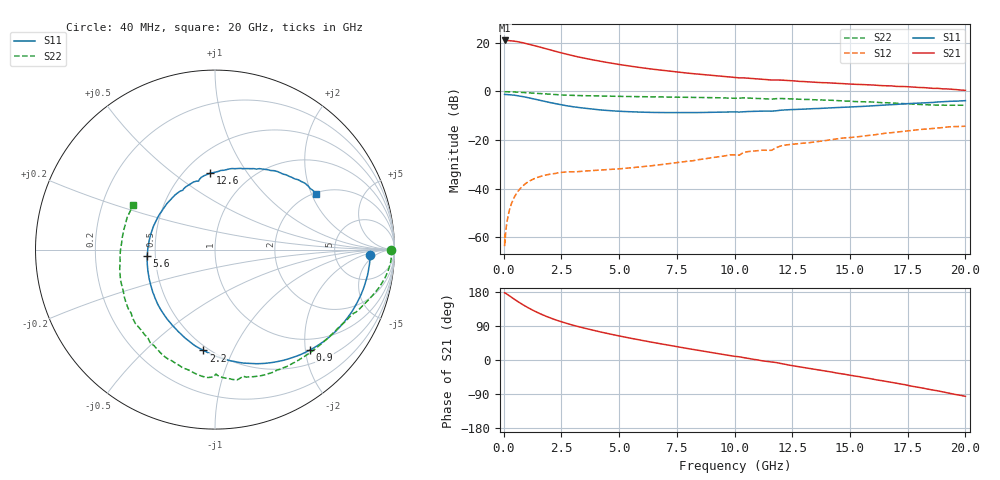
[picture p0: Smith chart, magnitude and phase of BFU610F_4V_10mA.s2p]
! Filename:  P:\Prog\Test\Noise\ATS_data\Testdata_Net\SplitFiles\BFU610_2W_A5_HighFreq_4V_10mA_D.s2p
! Date/Time: Wed 10/Aug/2011 16:57:59
! BFU610_2W_A5_HighFreq_4V_1mA_10mA_Bias4_R.s2p
! MDIF S-parameter v. bias file
! BFU610_2W_A5_HighFreq_4V_1mA_10mA
! Date/time Mon Aug 08 14:12:42 2011
! VAR V_out= 4.0010
! VAR I_out= 10.0000
! VAR V_in= 0.9022
! VAR I_in= 0.0905
! Device data file deembeded for feedlines and parallel
! Original file: \SplitFiles\BFU610_2W_A5_HighFreq_4V_10mA_R.s2p
! Feed-files: PR003V01_101208_Feed1.s2p, PR003V01_101208_Feed2.s2p
! Parallel-file: PR003V01_101208_Par.s2p
# MHz S MA R 50
!  Freq-MHz  S11-mag  S11-arg  S21-mag  S21-arg  S12-mag  S12-arg  S22-mag  S22-arg
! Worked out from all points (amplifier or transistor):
!   167 points, 40 MHz to 20 GHz, reference 50 ohm
!   highest |S21| = 21.0 dB at 40 MHz (marker M1)
!   |S21| within 3 dB of that: start of sweep to 1.673 GHz
!   unconditionally stable (mu >= 1): 3.031 GHz to end of sweep
!   at 550 MHz: K = 0.18, MSG = 31.3 dB, |S12| = -42.1 dB
!   at 4.2 GHz: K = 1.37, MAG = 18.8 dB, |S12| = -32.4 dB
!   at 20 GHz: K = 1.03, MAG = 6.4 dB, |S12| = -14.3 dB
!   S11 on the Smith chart (normalised r, x): 40 MHz: 13, -3; 900 MHz: 0.76, -2.10; 2.2 GHz: 0.47, -0.78; 5.6 GHz: 0.45, -0.04; 12.6 GHz: 0.66, +0.69; 20 GHz: 2.03, +2.17
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40  0.8651 -2.0  11.19 177.5  0.0006537 71.5  0.9812 0.0
50  0.8577 -2.6  11.14 177.5  0.001141 51.9  0.9827 -0.2
60  0.8669 -2.9  11.17 176.7  0.0007797 65.3  0.9836 -0.4
180  0.8616 -9.8  11.1 172.3  0.002616 81.8  0.9838 -2.4
400  0.8432 -21.6  10.91 162.9  0.005813 78.7  0.9768 -5.5
600  0.8179 -31.9  10.55 154.7  0.00855 73.0  0.9658 -8.2
900  0.7705 -46.5  9.864 143.4  0.01215 65.4  0.9455 -11.8
1150  0.7273 -57.8  9.226 134.9  0.01458 59.9  0.927 -14.5
1450  0.6761 -70.1  8.463 125.8  0.0169 54.3  0.9061 -17.3
1850  0.6133 -85.0  7.511 115.0  0.01915 48.5  0.8809 -20.6
2200  0.5657 -96.6  6.766 106.9  0.02037 45.0  0.8628 -23.5
2800  0.5001 -114.2  5.729 95.3  0.02221 39.9  0.8358 -27.3
3400  0.4571 -129.4  4.935 85.5  0.02267 39.4  0.8184 -31.3
4400  0.4081 -151.8  3.997 71.2  0.02436 40.0  0.8002 -37.8
5600  0.3793 -174.8  3.249 56.3  0.02701 43.7  0.7834 -45.9
6800  0.3674 165.1  2.738 42.7  0.03109 47.6  0.7704 -54.2
8800  0.3708 136.2  2.184 21.6  0.0416 51.2  0.7503 -68.7
10200  0.3763 118.5  1.904 8.4  0.0487 52.9  0.7254 -77.9
12600  0.426 93.8  1.643 -15.9  0.0825 43.4  0.6968 -99.7
13400  0.4421 85.8  1.55 -23.7  0.09037 38.9  0.6743 -107.4
16800  0.5342 56.3  1.3 -59.2  0.1417 16.1  0.578 -149.0
20000  0.6451 28.9  1.053 -95.8  0.1923 -16.9  0.5188 151.2
